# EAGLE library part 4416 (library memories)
DRAM 16K x 4 bits
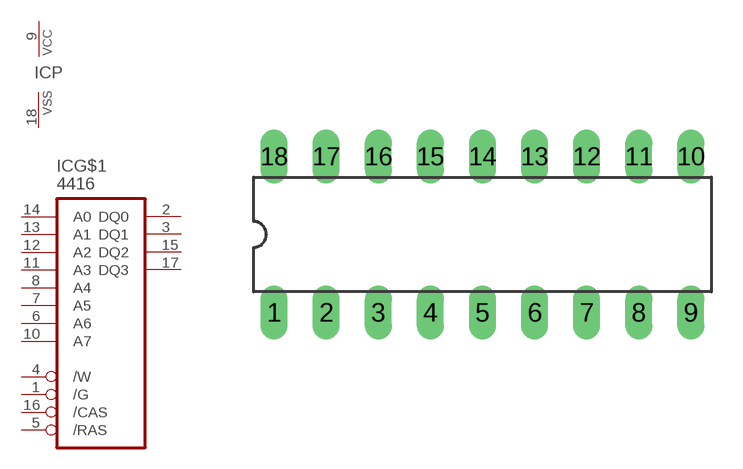
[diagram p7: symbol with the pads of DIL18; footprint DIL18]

Designator prefix IC; gates P=VCCVSS G$1=DRAM16KX4

## 4416  [DIL18]
1  G$1:/G  in
2  G$1:DQ0  out
3  G$1:DQ1  out
4  G$1:/W  in
5  G$1:/RAS  in
6  G$1:A6  in
7  G$1:A5  in
8  G$1:A4  in
9  P:VCC  pwr
10  G$1:A7  in
11  G$1:A3  in
12  G$1:A2  in
13  G$1:A1  in
14  G$1:A0  in
15  G$1:DQ2  out
16  G$1:/CAS  in
17  G$1:DQ3  out
18  P:VSS  pwr

## Footprint DIL18 (pad centres in mm)
Dual In Line
drill 0.813 long: 1 -10.16,-3.81; 2 -7.62,-3.81; 3 -5.08,-3.81; 4 -2.54,-3.81; 5 0,-3.81; 6 2.54,-3.81; 7 5.08,-3.81; 8 7.62,-3.81; 9 10.16,-3.81; 10 10.16,3.81; 11 7.62,3.81; 12 5.08,3.81; 13 2.54,3.81; 14 0,3.81; 15 -2.54,3.81; 16 -5.08,3.81; 17 -7.62,3.81; 18 -10.16,3.81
